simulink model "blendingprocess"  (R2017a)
settings: Solver=ode15s  StartTime=0.0  StopTime=3600.0  RelTol=1e-3  EnableMultiTasking=on

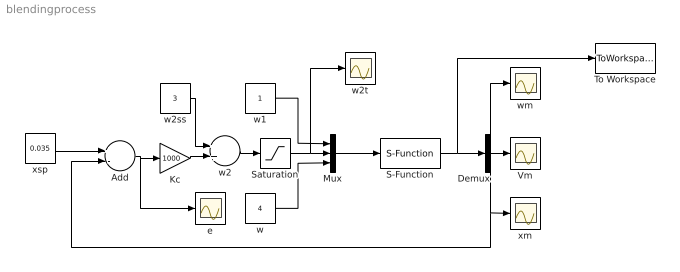
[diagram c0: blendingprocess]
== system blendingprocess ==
  Add : Sum  Inputs=+-
  Demux : Demux  Outputs=3
  Kc : Gain  Gain=1000
  Mux : Mux  Inputs=3
  S-Function : S-Function  FunctionName=sfunblend  SFunctionDeploymentMode=off  EnableBusSupport=off
  Saturation : Saturate  UpperLimit=10  LowerLimit=0
  To Workspace : ToWorkspace  VariableName=simout  SaveFormat=Timeseries  SampleTime=-1
  Vm : Scope
  e : Scope
  w : Constant  Value=4
  w1 : Constant
  w2 : Sum
  w2ss : Constant  Value=3
  w2t : Scope
  wm : Scope
  xm : Scope
  xsp : Constant  Value=0.035
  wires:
  S-Function/1 -> To Workspace/1, Demux/1
  Mux/1 -> S-Function/1
  w/1 -> Mux/3
  w1/1 -> Mux/1
  Demux/2 -> Vm/1
  Demux/1 -> wm/1
  Demux/3 -> Add/2, xm/1
  xsp/1 -> Add/1
  Add/1 -> e/1, Kc/1
  w2ss/1 -> w2/1
  Kc/1 -> w2/2
  w2/1 -> Saturation/1
  Saturation/1 -> w2t/1, Mux/2
